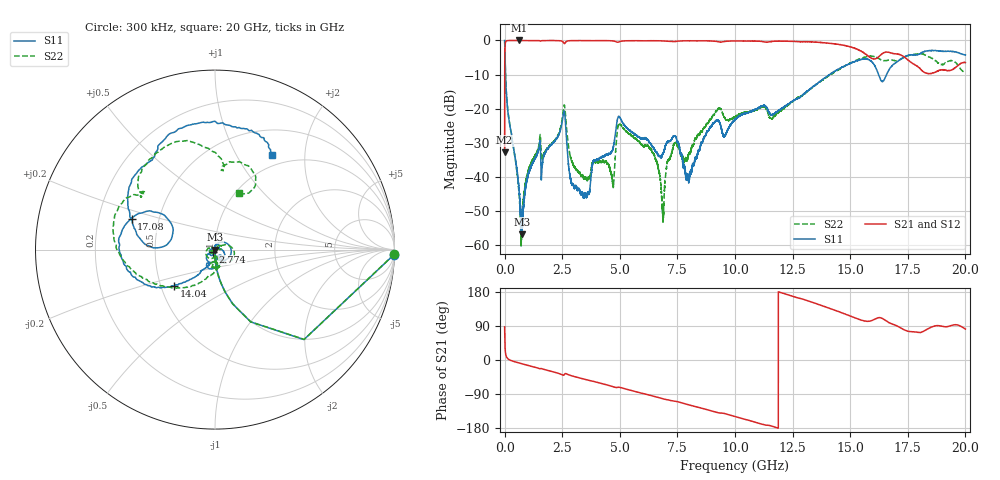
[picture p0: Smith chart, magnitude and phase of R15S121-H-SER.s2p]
!{R15S121}
!Johanson Technology Inc.
!www.johansontechnology.com
!Test Board Conditions:
!Substrate Type  RO4350B
!Substrate Thickness  20 mil
!Substrate Dk  3.66
!TL Type: GCPW
!TL Trace Width  34 mil
!TL Gap  10 mil
!Electrode orientation  Horizontal
!DUT TOPOLOGY	SERIES
!Mounting Pad LxW  26x52 mil
! Created Sat Feb  6 14:09:46 2021
# hz S ma R 50
! 2 Port Network Data from SP1.SP block
! freq  magS11  angS11  magS21  angS21  magS12  angS12  magS22  angS22
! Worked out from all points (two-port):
!   20001 points, 300 kHz to 20 GHz, reference 50 ohm
!   highest |S21| = 0.00 dB at 622.3 MHz (marker M1); lowest = -32.9 dB at 300 kHz (marker M2)
!   |S21| within 3 dB of the highest: 13.33 MHz to 15.42 GHz (15.41 GHz wide, 200 % of centre); 15.42634 GHz to 15.43427 GHz (7.929 MHz wide, 0.0514 % of centre)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
!   lowest |S11| = -56.9 dB at 741.3 MHz (marker M3), VSWR 1.00, Z = 49.9 - j0.00165 ohm
!   |S11| at or under -10 dB: 39.56 MHz to 14.11 GHz (14.07 GHz wide, 199 % of centre); 14.11132 GHz to 14.11277 GHz (1.455 MHz wide, 0.0103 % of centre); 16.23 GHz to 16.58 GHz (350.3 MHz wide, 2.14 % of centre)
!   |S22| runs from -60.4 to 0.0 dB; largest |S21 - S12| = 0.017
!   S11 on the Smith chart (normalised r, x): 300 kHz: 4, -72; 2.774 GHz: 0.98, -0.02; 14.04 GHz: 0.59, -0.26; 17.08 GHz: 0.35, +0.16; 20 GHz: 0.84, +1.41
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300000  0.9985 -1.6  0.02277 87.6  0.02276 88.3  0.9985 -1.5
1.083e8  0.1204 -84.5  0.9925 5.3  0.992 5.3  0.1205 -84.5
6.223e8  0.006958 -107.0  0.9999 -8.0  0.9976 -8.0  0.005933 -89.3
7.413e8  0.001426 -179.3  0.999 -10.0  0.9985 -10.0  0.001592 12.2
1.1233e9  0.01325 91.6  0.9983 -16.1  0.999 -16.1  0.01535 61.5
2.5433e9  0.07993 20.1  0.9452 -40.2  0.9453 -40.2  0.0932 8.1
2.7743e9  0.01481 -132.1  0.987 -38.9  0.9877 -38.9  0.02795 -74.6
3.3343e9  0.005743 159.2  0.9966 -48.6  0.9961 -48.6  0.01055 -69.3
4.6843e9  0.02435 -98.2  0.985 -70.1  0.9847 -70.0  0.008162 -145.0
4.9703e9  0.07618 -119.1  0.9542 -71.9  0.954 -72.0  0.05912 -131.6
6.6673e9  0.02048 -135.6  0.9898 -98.8  0.9902 -98.9  0.01332 141.2
6.8653e9  0.02155 -108.5  0.9836 -102.2  0.9841 -102.2  0.002936 176.1
7.3663e9  0.03953 -128.8  0.964 -108.5  0.9638 -108.5  0.03047 -140.2
7.9603e9  0.009432 100.6  0.9888 -117.7  0.9893 -117.7  0.02034 -120.8
8.9923e9  0.05652 -22.2  0.9812 -134.7  0.9806 -134.7  0.07362 -84.7
1.00003e10  0.06938 -53.7  0.9836 -149.2  0.9832 -149.2  0.07606 -80.1
1.33343e10  0.2031 -128.1  0.9522 152.7  0.9543 152.5  0.2003 -113.9
1.40443e10  0.3052 -138.3  0.9099 137.5  0.9186 137.5  0.2993 -134.5
1.66673e10  0.3608 177.1  0.6716 99.1  0.6559 99.3  0.5169 144.1
1.70763e10  0.4942 160.0  0.6292 88.5  0.6189 88.5  0.5105 142.2
1.84773e10  0.7104 99.5  0.327 85.4  0.3256 85.6  0.5641 93.7
2e10  0.6114 59.1  0.4739 81.6  0.4708 82.3  0.3434 67.1
